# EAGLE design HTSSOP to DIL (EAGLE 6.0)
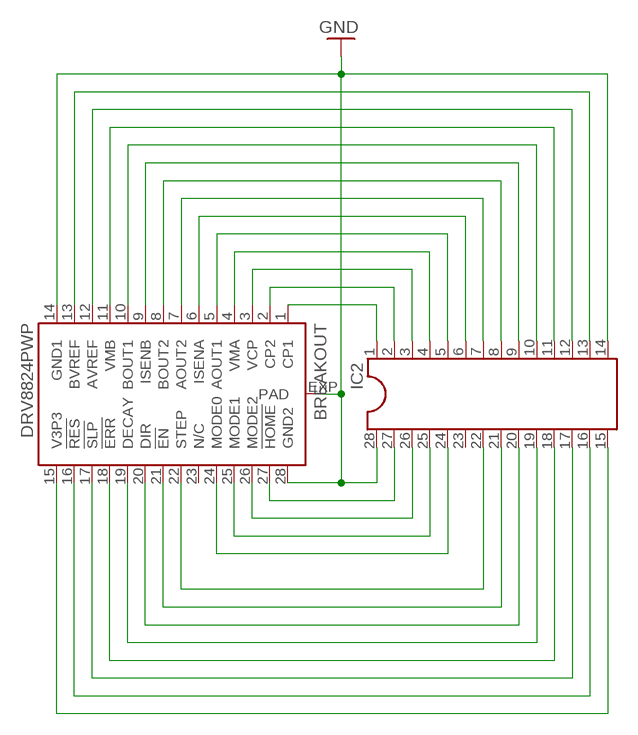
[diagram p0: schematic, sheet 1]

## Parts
BREAKOUT  DRV8824PWP  [HTSSOP28PWP]
IC2  DIL28  [DIL28-6]

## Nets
!EN: BREAKOUT.21(!EN) IC2.21
!ERR: BREAKOUT.18(!ERR) IC2.18
!HOME: BREAKOUT.27(!HOME) IC2.27
!RES: BREAKOUT.16(!RES) IC2.16
!SLP: BREAKOUT.17(!SLP) IC2.17
AOUT1: BREAKOUT.5(AOUT1) IC2.5
AOUT2: BREAKOUT.7(AOUT2) IC2.7
AVREF: BREAKOUT.12(AVREF) IC2.12
BOUT1: BREAKOUT.10(BOUT1) IC2.10
BOUT2: BREAKOUT.8(BOUT2) IC2.8
BVREF: BREAKOUT.13(BVREF) IC2.13
CP1: BREAKOUT.1(CP1) IC2.1
CP2: BREAKOUT.2(CP2) IC2.2
DECAY: BREAKOUT.19(DECAY) IC2.19
DIR: BREAKOUT.20(DIR) IC2.20
GND: BREAKOUT.14(GND1) BREAKOUT.28(GND2) BREAKOUT.EXP(PAD) IC2.14 IC2.28
ISENA: BREAKOUT.6(ISENA) IC2.6
ISENB: BREAKOUT.9(ISENB) IC2.9
MODE0: BREAKOUT.24(MODE0) IC2.24
MODE1: BREAKOUT.25(MODE1) IC2.25
MODE2: BREAKOUT.26(MODE2) IC2.26
STEP: BREAKOUT.22(STEP) IC2.22
V3P3: BREAKOUT.15(V3P3) IC2.15
VCP: BREAKOUT.3(VCP) IC2.3
VMA: BREAKOUT.4(VMA) IC2.4
VMB: BREAKOUT.11(VMB) IC2.11
Unconnected: BREAKOUT.23(N/C) IC2.23

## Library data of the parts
BREAKOUT = texas:DRV8824
IC2 = ic-package:DIL28: Dual In Line

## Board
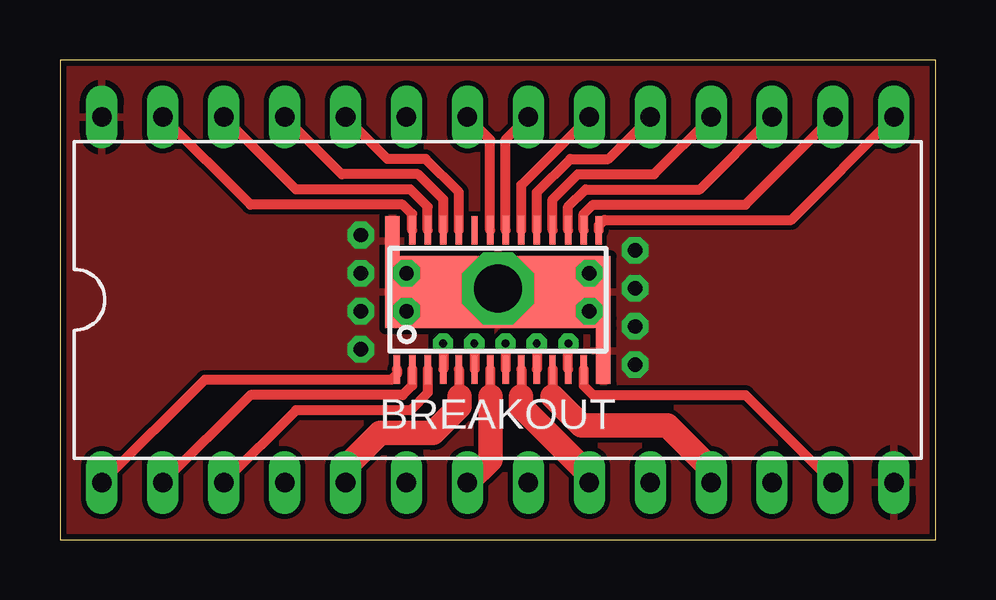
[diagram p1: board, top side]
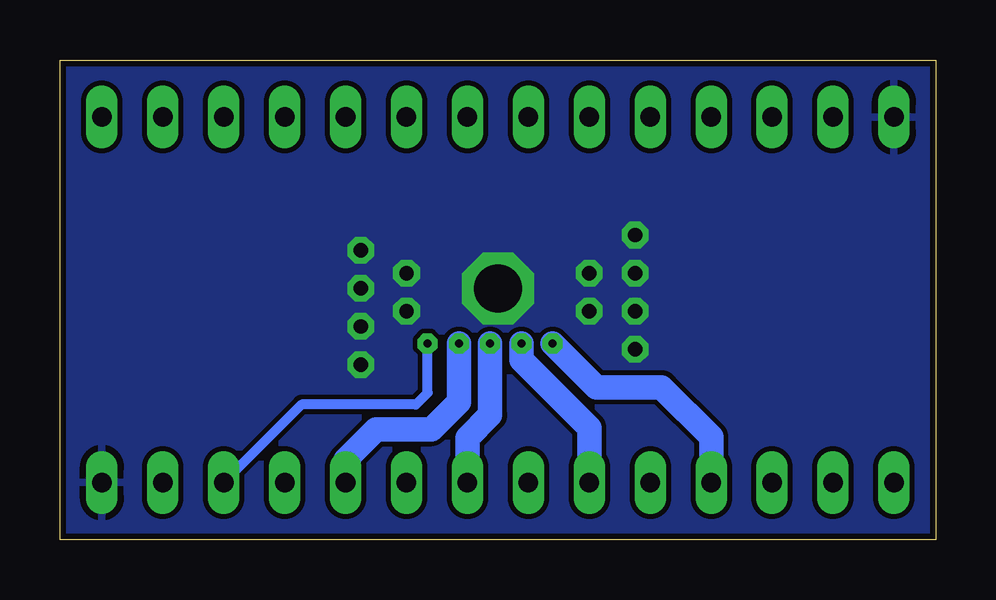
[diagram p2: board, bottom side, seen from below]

Size 36.51 x 20 mm. Coordinates in mm from the lower left corner, seen from the top.
Outline: 0,0 36.51,0 36.51,20 0,20 0,0
Copper layers (1*16): Top 0.035mm / dielectric 1.5mm / Bottom 0.035mm
Design rules: minimum track width 0.2mm, minimum drill 13mil, track to track 0.2mm, track to pad 0.2mm, pad to pad 0.2mm, via to via 0.2mm, smd to smd 0mil, copper to edge 10mil, drill to drill 0.2mm, minimum pad ring 10mil, minimum via ring 10mil, stop-mask expansion 0.125mm, vias tented up to drill 20mil, thermal gap 10mil

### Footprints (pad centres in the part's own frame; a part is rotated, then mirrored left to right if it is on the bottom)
HTSSOP28PWP = smd 0.27 x 1.2: 1 -4.21,-2.9; 2 -3.575,-2.9; 3 -2.925,-2.9; 4 -2.275,-2.9; 5 -1.625,-2.9; 6 -0.975,-2.9; 7 -0.325,-2.9; 8 0.325,-2.9; 9 0.975,-2.9; 10 1.625,-2.9; 11 2.275,-2.9; 12 2.925,-2.9; 13 3.575,-2.9; 15 4.21,2.9; 16 3.575,2.9; 17 2.925,2.9; 18 2.275,2.9; 19 1.625,2.9; 20 0.975,2.9; 21 0.325,2.9; 22 -0.325,2.9; 23 -0.975,2.9; 24 -1.625,2.9; 25 -2.275,2.9; 26 -2.925,2.9; 27 -3.575,2.9 | smd 0.61 x 2.735: 14 4.395,-2.132 | smd 0.61 x 2.1: 28 -4.395,2.45 | smd 9.4 x 3: EXP 0,0.318
DIL28-6 = drill 0.813 long: 1 -16.51,-7.62; 2 -13.97,-7.62; 3 -11.43,-7.62; 4 -8.89,-7.62; 5 -6.35,-7.62; 6 -3.81,-7.62; 7 -1.27,-7.62; 8 1.27,-7.62; 9 3.81,-7.62; 10 6.35,-7.62; 11 8.89,-7.62; 12 11.43,-7.62; 13 13.97,-7.62; 14 16.51,-7.62; 15 16.51,7.62; 16 13.97,7.62; 17 11.43,7.62; 18 8.89,7.62; 19 6.35,7.62; 20 3.81,7.62; 21 1.27,7.62; 22 -1.27,7.62; 23 -3.81,7.62; 24 -6.35,7.62; 25 -8.89,7.62; 26 -11.43,7.62; 27 -13.97,7.62; 28 -16.51,7.62

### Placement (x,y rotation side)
BREAKOUT  18.26,10 0 top
IC2  18.26,10 0 top

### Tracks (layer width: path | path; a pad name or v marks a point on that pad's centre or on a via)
!EN
  Top 0.406: BREAKOUT.21 18.58,16.68 IC2.21
!ERR
  Top 0.406: BREAKOUT.18 20.53,14.18 21.59,15.24 24.77,15.24 IC2.18
!HOME
  Top 0.406: BREAKOUT.27 14.68,13.58 14.29,13.97 7.94,13.97 IC2.27
!RES
  Top 0.406: BREAKOUT.16 21.83,13.58 22.23,13.97 28.57,13.97 IC2.16
!SLP
  Top 0.406: BREAKOUT.17 21.18,13.88 21.91,14.61 26.67,14.61 IC2.17
AOUT1
  Top 0.406: 11.91,3.02 IC2.5 | BREAKOUT.5 16.63,6.19 16.66,5.97
  Top 1.016: 11.91,3.02 13.34,4.45 15.56,4.45 16.66,5.56 16.66,5.97
AOUT2
  Top 0.406: BREAKOUT.7 17.93,6.44 17.94,5.97
  Top 1.016: 17.94,5.97 17.94,3.33 IC2.7
AVREF  (via drill 0.33)
  Top 0.406: BREAKOUT.12 21.18,8.16 v21.19,8.18
  Bottom 0.406: IC2.12 26.43,5.64 21.67,5.64 21.18,6.12 21.18,8.16 v21.19,8.18
BOUT1  (via drill 0.33)
  Top 0.406: v19.88,8.18 BREAKOUT.10
  Bottom 1.016: IC2.10 24.61,3.33 23.34,4.6 21.03,4.6 19.88,5.75 v19.88,8.17 v19.88,8.18
BOUT2  (via drill 0.33)
  Top 0.406: v18.58,8.18 BREAKOUT.8
  Bottom 1.016: IC2.8 19.53,4.25 18.58,5.2 v18.58,8.17 v18.58,8.18
BVREF
  Top 0.406: BREAKOUT.13 21.83,6.43 22.23,6.03 28.57,6.03 IC2.13
CP1
  Top 0.406: BREAKOUT.1 14.05,6.9 13.81,6.67 6.03,6.67 IC2.1
CP2
  Top 0.406: BREAKOUT.2 14.68,6.43 14.29,6.03 7.94,6.03 IC2.2
DECAY
  Top 0.406: BREAKOUT.19 19.88,14.48 21.27,15.88 22.86,15.88 IC2.19
DIR
  Top 0.406: BREAKOUT.20 19.23,14.79 IC2.20
GND  (via drill 0.6, 2)
  other vias: 18.26,10.48 12.54,12.7 12.54,11.11 12.54,9.53 12.54,7.94 23.97,7.3 23.97,8.89 23.97,10.48 23.97,12.06 22.07,9.53 22.07,11.11 14.45,11.11 14.45,9.53
  pour Top: 0,20 0,0 36.51,0 36.51,20
  pour Bottom: 0,20 0,0 36.51,0 36.51,20
ISENA  (via drill 0.33)
  Top 0.406: v17.27,8.18 v17.28,8.18 BREAKOUT.6
  Bottom 1.016: IC2.6 14.45,4.66 17.28,7.5 17.28,8.17 v17.27,8.18
ISENB
  Top 0.406: 22.07,2.7 IC2.9 | BREAKOUT.9 19.23,5.87 19.21,5.97
  Top 1.016: 22.07,2.7 19.21,5.56 19.21,5.97
MODE0
  Top 0.406: BREAKOUT.24 16.63,14.48 15.24,15.88 13.65,15.88 IC2.24
MODE1
  Top 0.406: BREAKOUT.25 15.98,14.18 14.92,15.24 11.75,15.24 IC2.25
MODE2
  Top 0.406: BREAKOUT.26 15.33,13.88 14.61,14.61 9.84,14.61 IC2.26
STEP
  Top 0.406: BREAKOUT.22 17.93,16.68 IC2.22
V3P3
  Top 0.406: BREAKOUT.15 22.47,13.1 22.7,13.34 30.48,13.34 IC2.15
VCP
  Top 0.406: BREAKOUT.3 15.33,6.12 14.61,5.4 9.84,5.4 IC2.3
VMA  (via drill 0.33)
  Top 0.406: v15.98,8.18 BREAKOUT.4
  Bottom 1.016: IC2.4 9.37,4.29 11.43,6.35 14.15,6.35 v15.98,8.18
VMB
  Top 0.406: BREAKOUT.11 20.53,5.97 | 27.15,2.94 IC2.11
  Top 1.016: 20.53,5.97 21.74,4.76 25.32,4.76 27.15,2.94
